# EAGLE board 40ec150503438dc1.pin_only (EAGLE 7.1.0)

Size 12.7 x 20.32 mm. Coordinates in mm from the lower left corner, seen from the top.
Outline: 12.7,20.32 0,20.32 0,0 12.7,0 12.7,20.32
Copper layers (1*16): Top 0.035mm / dielectric 1.5mm / Bottom 0.035mm
Design rules "SparkFun-2-layer": minimum track width 7mil, minimum drill 15mil, track to track 8mil, track to pad 8mil, pad to pad 8mil, via to via 8mil, smd to smd 8mil, copper to edge 8mil, drill to drill 8mil, minimum pad ring 12mil, minimum via ring 10mil, stop-mask expansion 4mil, vias tented up to drill 20mil, thermal gap 10mil

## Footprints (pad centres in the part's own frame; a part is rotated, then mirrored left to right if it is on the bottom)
0603-CAP = smd 1.1 x 1: 1 -0.85,0; 2 0.85,0
FIDUCIAL-1X2 = smd 1 x 1: 1 0,0
1X04_NO_SILK = drill 1.016 pad 1.88 square: 1 0,0 | drill 1.016 pad 1.88: 2 2.54,0; 3 5.08,0; 4 7.62,0
1X06_NO_SILK = drill 1.016 pad 1.88: 1 0,0; 2 2.54,0; 3 5.08,0; 4 7.62,0; 5 10.16,0; 6 12.7,0
0603-RES = smd 1.1 x 1: 1 -0.85,0; 2 0.85,0
PAD-JUMPER-3-3OF3_NC_BY_TRACE_YES_SILK_FULL_BOX = smd 0.635 x 1.27: 1 -0.813,0; 2 0,0; 3 0.813,0
PAD-JUMPER-2-NC_BY_TRACE_YES_SILK = smd 0.635 x 1.27: 1 -0.508,0; 2 0.508,0
PAD-JUMPER-3-2OF3_NC_BY_TRACE_YES_SILK_FULL_BOX = smd 0.635 x 1.27: 1 -0.813,0; 2 0,0; 3 0.813,0
STAND-OFF = hole 3.302: 0,0
BME280_LGA = smd 0.5 x 0.35: P$1 1.025,0.975; P$2 1.025,0.325; P$3 1.025,-0.325; P$4 1.025,-0.975; P$5 -1.025,-0.975; P$6 -1.025,-0.325; P$7 -1.025,0.325; P$8 -1.025,0.975

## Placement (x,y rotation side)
C1  0.1uF  [0603-CAP]  7.62,15.8 0 top
C2  0.1uF  [0603-CAP]  7.62,14.21 180 top
FID1  FIDUCIAL1X2  [FIDUCIAL-1X2]  3.81,19.37 0 top
FID2  FIDUCIAL1X2  [FIDUCIAL-1X2]  8.57,0.87 0 top
FRAME1  FRAME-LETTER  [CREATIVE_COMMONS]  not placed on the board
JP1  [1X04_NO_SILK]  1.27,17.78 270 top
JP2  [1X06_NO_SILK]  11.43,5.08 90 top
LOGO1  SFE_LOGO_FLAME.1_INCH  [SFE_LOGO_FLAME_.1]  7.46,10 0 bottom
LOGO2  SFE_LOGO_FLAME.1_INCH  [SFE_LOGO_FLAME_.1]  3.89,4.13 0 top
LOGO3  OSHW-LOGOS  [OSHW-LOGO-S]  10.48,1.91 0 top
R1  4.7K  [0603-RES]  2.54,6.99 180 top
R2  4.7K  [0603-RES]  2.54,5.71 180 top
R3  4.7K  [0603-RES]  7.94,6.99 0 top
R4  4.7K  [0603-RES]  7.3,17.78 0 top
SJ1  EN I2C PULL  [PAD-JUMPER-3-3OF3_NC_BY_TRACE_YES_SILK_FULL_BOX]  3.17,6.35 90 bottom
SJ2  EN I2C MODE  [PAD-JUMPER-2-NC_BY_TRACE_YES_SILK]  7.3,6.67 270 bottom
SJ3  EN ADR PULLUP  [PAD-JUMPER-3-2OF3_NC_BY_TRACE_YES_SILK_FULL_BOX]  4.76,19.05 180 bottom
STANDOFF4  STAND-OFF  [STAND-OFF]  6.35,2.54 0 top
U1  BME280  [BME280_LGA]  6.35,11.43 270 top

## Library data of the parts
C1 C2 = SparkFun-Capacitors; PROD_ID: CAP-08604
FID1 FID2 FRAME1 LOGO1-LOGO3 = SparkFun-Aesthetics
JP1 = SparkFun-Connectors
JP2 = SparkFun-Connectors; PROD_ID: CONN-08437
R1-R4 = SparkFun-Resistors; PROD_ID: RES-07857
SJ1-SJ3 = SparkFun-Passives
STANDOFF4 = SparkFun-Electromechanical
U1 = BME280ComponentLibrary; PROD_ID: IC-13090

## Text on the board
Bottom: v10
tPlace: GND | GND | 3.3V | 3.3V | SCK | SDA | SCL | SDO | SDI | !CS | BME / 280
bPlace: 0 | 1 | ADR: | GND | GND | 3.3 | 3.3V | SDA | SCK | SCL | SDO | CS / PU | SDI | !CS | I2C / PU
Measures: Units in inches
tDocu: Marshall Taylor | Note: Top and bottom ground planes must be isolated / no more than 0.008 inch to allow proper grounding.

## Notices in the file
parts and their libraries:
SparkFun-Capacitors: Licensing: Creative Commons ShareAlike 4.0 International - https://creativecommons.org/licenses/by-sa/4.0
SparkFun-Aesthetics: Released under the Creative Commons Attribution Share-Alike 4.0 License
SparkFun-Aesthetics: https://creativecommons.org/licenses/by-sa/4.0
